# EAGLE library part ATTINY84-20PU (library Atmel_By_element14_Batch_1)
8-bit Microcontroller with In-System Programmable Flash
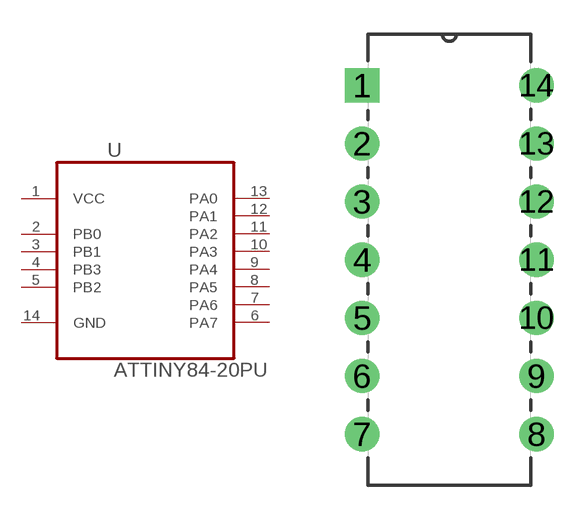
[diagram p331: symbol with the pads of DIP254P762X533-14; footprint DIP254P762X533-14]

Designator prefix U

## ATTINY84-20PU (MPN: ATTINY84-20PU; OC_FARNELL: -; OC_NEWARK: 58M3794; PACKAGE: PDIP-14; SUPPLIER: Atmel)  [DIP254P762X533-14]
1  VCC  pwr
2  PB0
3  PB1
4  PB3
5  PB2
6  PA7
7  PA6
8  PA5
9  PA4
10  PA3
11  PA2
12  PA1
13  PA0
14  GND  pas

## Footprint DIP254P762X533-14 (pad centres in mm)
drill 0.991 square: 1 -7.62,15.24
drill 0.991: 2 -7.62,12.7; 3 -7.62,10.16; 4 -7.62,7.62; 5 -7.62,5.08; 6 -7.62,2.54; 7 -7.62,0; 8 0,0; 9 0,2.54; 10 0,5.08; 11 0,7.62; 12 0,10.16; 13 0,12.7; 14 0,15.24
